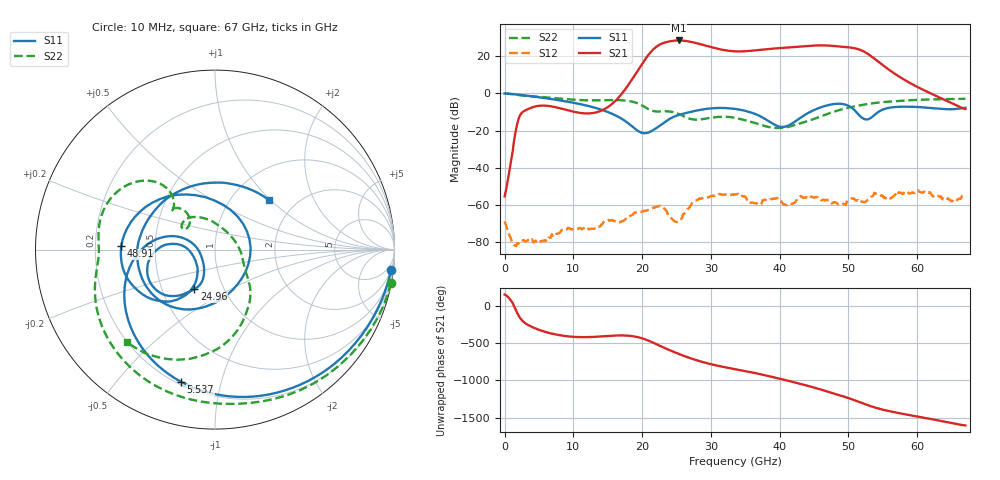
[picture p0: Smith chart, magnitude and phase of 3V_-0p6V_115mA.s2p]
! MARKI MICROWAVE INC.
! Date:  10/23/18
! Model Number:  AMM-6702CH
! Description:  2-port Small Signal S-parameter data for AMM-6702CH
! Frequency Range:  10 MHz to 67 GHz
! Port Configuration:  PORT 1: Input
!  PORT 2: Output
! Bias Condition: Vd = +3V, Vg = -0.6V
! AMM-6702CH s2p files are only valid for small signal conditions (below -5 dBm input power)
!S2P File: Measurements: Mag<S11> Ang<S11>, Mag<S21> Ang<S21>, Mag<S12> Ang<S12>, Mag<S22> Ang<S22>!row 1
# Hz S  dB  R 50
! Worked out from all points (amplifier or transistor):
!   401 points, 10 MHz to 67 GHz, reference 50 ohm
!   highest |S21| = 28.4 dB at 25.3 GHz (marker M1)
!   |S21| within 3 dB of that: 22.23 GHz to 29.44 GHz (7.207 GHz wide, 27.9 % of centre)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
!   unconditionally stable (mu >= 1): start of sweep to end of sweep
!   at 11.06 GHz: K = 2991.97, MAG = -6.8 dB, |S12| = -72.5 dB
!   at 33.51 GHz: K = 15.71, MAG = 23.5 dB, |S12| = -54.3 dB
!   at 67 GHz: K = 271.82, MAG = -4.6 dB, |S12| = -54.0 dB
!   S11 on the Smith chart (normalised r, x): 10 MHz: 2, -17; 5.537 GHz: 0.22, -0.75; 24.96 GHz: 0.73, -0.34; 48.91 GHz: 0.31, +0.02; 67 GHz: 1.48, +0.98
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1e7  -0.11 -6.7  -55.42 158.2  -68.90 -29.9  -0.02 -10.8
5.536675e9  -2.38 -104.4  -6.60 26.0  -79.22 -147.0  -2.01 -133.0
1.123082e10  -5.99 -165.4  -10.64 -56.2  -73.13 148.9  -3.67 -174.2
1.993952e10  -21.22 -169.8  15.50 -70.0  -63.73 132.4  -6.40 129.8
2.14468e10  -20.12 -131.6  22.93 -123.8  -61.92 120.2  -9.32 131.9
2.245165e10  -17.71 -117.8  25.95 -167.8  -60.65 98.0  -9.80 138.0
2.362398e10  -14.68 -112.2  27.64 142.8  -63.78 64.4  -9.65 136.6
2.496378e10  -12.07 -117.6  28.39 91.2  -69.19 116.7  -10.61 129.7
2.529872e10  -11.66 -119.5  28.43 78.9  -68.97 131.3  -11.07 128.4
2.647105e10  -10.53 -124.4  28.10 37.9  -62.95 131.3  -13.04 129.5
2.764338e10  -9.51 -129.7  27.22 0.9  -57.83 111.0  -14.14 138.6
2.998802e10  -8.12 -143.4  24.88 -60.0  -55.27 103.2  -13.16 146.9
3.3505e10  -8.39 -168.7  22.57 -127.2  -54.32 36.7  -13.19 124.1
3.735692e10  -12.66 172.1  23.44 161.0  -59.38 40.3  -17.07 84.7
4.053895e10  -18.08 -151.9  24.47 91.5  -59.72 33.8  -18.52 28.1
4.472582e10  -9.44 -126.0  25.62 -8.6  -55.65 13.7  -14.12 -32.5
4.6903e10  -6.48 -148.3  25.71 -68.4  -57.23 -30.7  -11.16 -45.8
4.89127e10  -5.64 178.0  25.10 -125.3  -59.71 -59.2  -8.73 -59.3
5.058745e10  -8.05 131.4  24.44 -176.4  -56.62 -29.3  -7.24 -69.7
5.22622e10  -13.77 29.3  22.43 125.6  -58.52 167.4  -6.06 -79.3
5.594665e10  -7.74 -132.3  12.56 26.2  -57.16 59.4  -4.45 -97.9
6.7e10  -7.76 42.3  -8.45 -166.4  -54.01 -133.8  -2.94 -133.5
